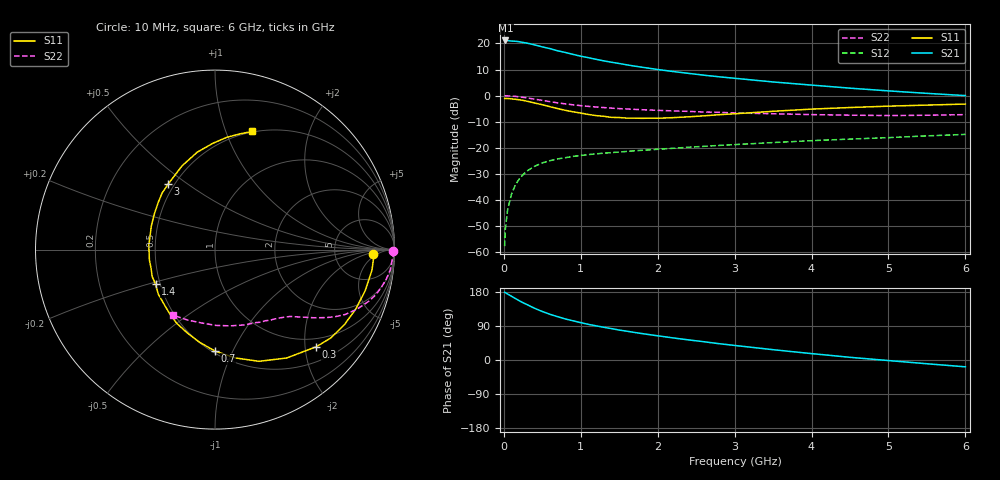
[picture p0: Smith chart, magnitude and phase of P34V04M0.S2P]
! SIEMENS Small Signal Semiconductors
! BFP181
! Si NPN RF Bipolar Junction Transistor in SOT143
! VCE = 4 V  IC = 4 mA
! Common Emitter S-Parameters:  March  1996
# GHz  S  MA  R  50
!  f  S11  S21  S12  S22
! GHz  MAG  ANG  MAG  ANG  MAG  ANG  MAG  ANG
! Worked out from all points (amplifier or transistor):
!   36 points, 10 MHz to 6 GHz, reference 50 ohm
!   highest |S21| = 21.2 dB at 20 MHz (marker M1)
!   |S21| within 3 dB of that: start of sweep to 580.5 MHz
!   unconditionally stable (mu >= 1): 1.897 GHz to end of sweep
!   at 250 MHz: K = 0.18, MSG = 25.3 dB, |S12| = -30.3 dB
!   at 1.4 GHz: K = 0.84, MSG = 17.3 dB, |S12| = -21.8 dB
!   at 6 GHz: K = 1.06, MAG = 5.9 dB, |S12| = -14.9 dB
!   S11 on the Smith chart (normalised r, x): 10 MHz: 15, -3; 300 MHz: 0.80, -2.24; 700 MHz: 0.52, -0.86; 1.4 GHz: 0.47, -0.21; 3 GHz: 0.46, +0.42; 6 GHz: 0.49, +1.24
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0.01  0.882 -1.5  11.38 178.7  0.0013 84.8  0.9926 -0.6
0.02  0.8845 -3.2  11.43 177.9  0.0028 81.8  0.9952 -1.4
0.05  0.8821 -7.4  11.35 173.9  0.0066 86.4  0.9886 -3.4
0.1  0.8679 -15.1  11.12 168.2  0.0129 79.5  0.9827 -6.7
0.15  0.8515 -22.9  11.03 162.2  0.0194 76.2  0.9676 -9.9
0.2  0.8335 -30.1  10.8 156.5  0.0252 73.5  0.9496 -12.9
0.3  0.7816 -43.9  10.18 146.4  0.0359 66.2  0.9058 -18.4
0.4  0.7236 -56.6  9.408 136.4  0.0442 60.6  0.8576 -22.8
0.5  0.669 -68.5  8.604 128.0  0.0514 55.1  0.8116 -26.4
0.6  0.6133 -79.6  7.976 120.6  0.0567 51.1  0.7665 -29.2
0.7  0.565 -90.0  7.241 114.3  0.0613 48.1  0.7269 -31.4
0.8  0.5229 -99.6  6.718 108.3  0.0646 45.6  0.6949 -33.1
0.9  0.49 -108.2  6.184 103.4  0.0685 43.0  0.6669 -34.7
1.1  0.4355 -125.8  5.34 94.0  0.0741 40.4  0.6227 -37.2
1.4  0.3833 -149.8  4.368 82.8  0.0809 37.4  0.5765 -40.4
1.8  0.3675 -177.7  3.503 69.6  0.0897 35.4  0.5371 -44.6
2.2  0.3785 159.6  2.9 58.3  0.0979 33.9  0.5095 -49.3
3  0.4487 125.6  2.153 38.4  0.1151 30.6  0.4662 -60.7
3.5  0.5014 111.5  1.83 27.2  0.1261 28.3  0.4497 -69.1
4.5  0.5921 91.2  1.392 7.1  0.1469 22.6  0.4223 -89.4
5.5  0.6591 77.9  1.106 -9.9  0.1693 17.7  0.421 -111.1
6  0.6897 72.6  1.002 -18.0  0.1807 14.4  0.4329 -122.3
